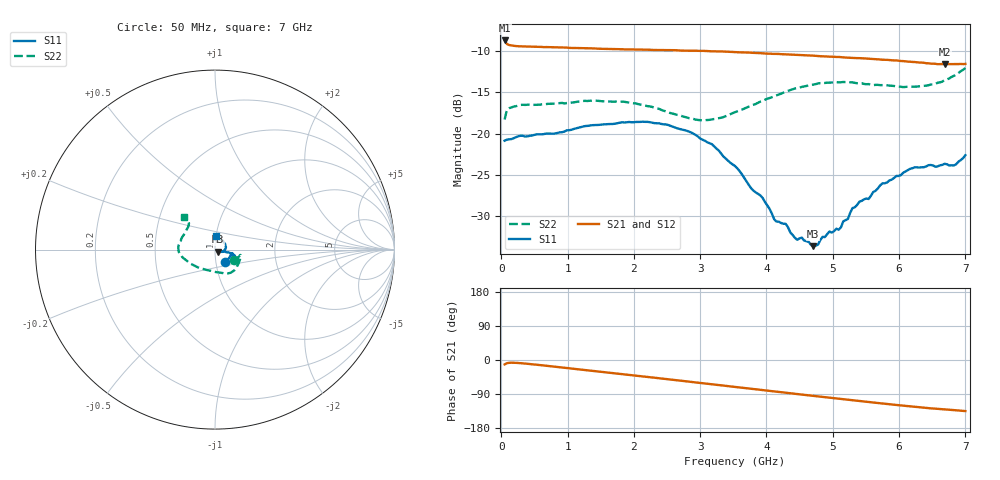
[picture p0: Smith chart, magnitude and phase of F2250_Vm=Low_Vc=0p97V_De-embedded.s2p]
! Integrated Device Technology
! Corporate Headquarters
! 6024 Silver Creek Valley Road
! San Jose, CA 95138  USA
! Phone:  1-408-284-8200
! Toll Free:  1-800-223-1366
! Webpage:  http://www.idt.com/
! Timing and RF Division
! 515 Groton Road, Suite 102
! Westford, MA 01886-6024
! Device:  F2250
! Description: Voltage Variable RF Attenuator
! Frequency:  50.0 -  6000.00 MHz
! Package:  3x3 mm Thin QFN Plastic Package: 16 pin
! Ports:  2 RF, 3 DC
!  Pin  1  = GND
!  Pin  2  = NC
!  Pin  3  = RF1  = Port 1
!  Pin  4  = NC
!  Pin  5  = GND
!  Pin  6  = GND
!  Pin  7  = GND
!  Pin  8  = GND
!  Pin  9  = NC
!  Pin 10  = RF2  = Port 2
!  Pin 11  = NC
!  Pin 12  = GND
!  Pin 13  = GND
!  Pin 14  = VCNTRL
!  Pin 15  = VDD
!  Pin 16  = VMODE
! Vcntrl:  0.970 Volts
! Vmode:  +0.000 Volts
! Vdd:  +3.30  Volts
! Current:  1.183 mA
! Data:  The device was measured on a the F2250 evaluation board which has
!  individual transmission lines to the RF pins.  Data was collected
!  using a calibrated network analyzer.  The evaluation board was
!  de-embedded using a TRL calibration technique.
!  The reference plane is the edge of the package pin.
! Misc:  SN 10
!  Action Tracker AT0258
! Date Measured:  2014-11-26
! Date:  2015-10-15  MJV
! Note:
!  Integrated Device Technology supplies this data as a sample of measured
!  data at the package pin for this product.  Your particular data for this
!  product may vary.
!  Data was taken at 25 degrees C.
!  Integrated Device Technology reserves the right to change this data at anytime.
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# GHz S dB R 50
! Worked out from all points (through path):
!   201 points, 50 MHz to 7 GHz, reference 50 ohm
!   highest |S21| = -8.73 dB at 50 MHz (marker M1); lowest = -11.6 dB at 6.687 GHz (marker M2)
!   group delay of S21, straight-line fit = 53.8 ps
!   lowest |S11| = -33.6 dB at 4.707 GHz (marker M3), VSWR 1.04, Z = 51.8 - j1.13 ohm
!   |S11| at or under -10 dB: start of sweep to end of sweep
!   |S22| runs from -18.4 to -12.1 dB; largest |S21 - S12| = 0.00082
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0.05  -20.85 -52.3  -8.73 -11.6  -8.74 -11.7  -18.29 -29.7
0.08475  -20.72 -28.3  -9.16 -8.5  -9.15 -8.5  -17.11 -16.3
0.29325  -20.25 -11.8  -9.44 -8.4  -9.44 -8.4  -16.53 -14.2
1.2315  -19.15 -20.9  -9.66 -25.9  -9.65 -25.9  -16.05 -41.8
2.37825  -18.76 -17.4  -9.89 -48.1  -9.89 -48.1  -17.00 -69.5
3.0385  -20.75 -13.2  -9.98 -61.3  -9.99 -61.3  -18.40 -101.4
3.525  -23.92 -13.0  -10.13 -71.1  -10.15 -71.1  -17.41 -131.1
3.942  -27.78 -15.8  -10.28 -79.5  -10.29 -79.5  -16.02 -151.0
4.11575  -30.36 -17.6  -10.35 -83.0  -10.34 -83.0  -15.48 -158.0
4.2895  -30.91 -24.9  -10.40 -86.4  -10.40 -86.4  -14.92 -163.5
4.46325  -32.85 -28.7  -10.47 -89.9  -10.49 -89.9  -14.51 -168.2
4.53275  -32.59 -28.1  -10.50 -91.3  -10.50 -91.3  -14.34 -170.3
4.7065  -33.62 -31.6  -10.56 -94.7  -10.57 -94.7  -14.07 -174.1
4.94975  -31.84 -29.9  -10.69 -99.4  -10.67 -99.5  -13.83 -179.3
5.08875  -31.63 -26.5  -10.72 -102.2  -10.72 -102.2  -13.79 177.5
5.22775  -30.32 -25.2  -10.81 -104.8  -10.79 -104.8  -13.78 174.5
5.29725  -29.01 -21.8  -10.83 -106.1  -10.84 -106.1  -13.81 172.9
5.85325  -25.67 -4.8  -11.10 -116.7  -11.10 -116.8  -14.20 158.4
6.2355  -24.08 12.9  -11.34 -123.6  -11.34 -123.7  -14.32 145.9
6.68725  -23.65 47.4  -11.61 -130.3  -11.61 -130.4  -13.52 134.2
6.82625  -23.85 61.7  -11.58 -132.2  -11.60 -132.2  -13.01 134.0
7  -22.61 85.9  -11.57 -134.8  -11.56 -134.9  -12.06 133.9
